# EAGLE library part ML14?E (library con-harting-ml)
HARTING
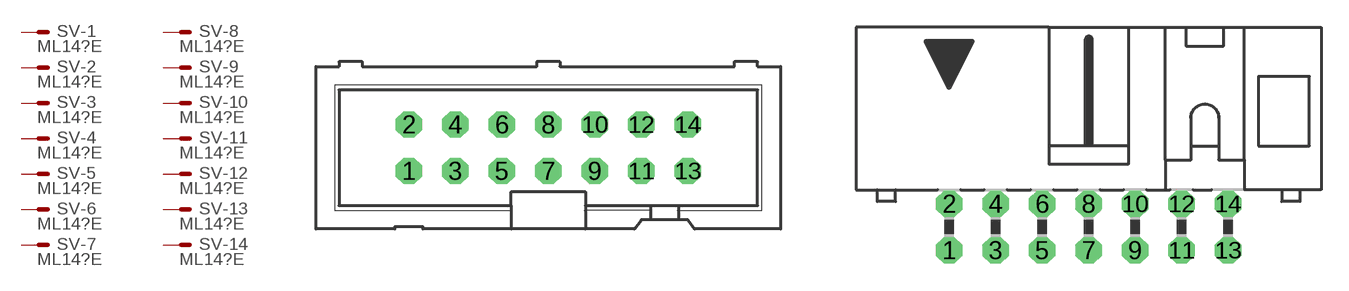
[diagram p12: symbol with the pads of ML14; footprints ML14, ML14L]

Designator prefix SV; gates -1=M -2=M -3=M -4=M -5=M -6=M -7=M -8=M -9=M -10=M -11=M -12=M -13=M -14=M

## ML14E (OC_FARNELL: unknown; OC_NEWARK: unknown)  [ML14]
1  -1:S  pas
2  -2:S  pas
3  -3:S  pas
4  -4:S  pas
5  -5:S  pas
6  -6:S  pas
7  -7:S  pas
8  -8:S  pas
9  -9:S  pas
10  -10:S  pas
11  -11:S  pas
12  -12:S  pas
13  -13:S  pas
14  -14:S  pas

## ML14LE (OC_FARNELL: unknown; OC_NEWARK: unknown)  [ML14L]
Pads as for ML14

## ML143ME (OC_FARNELL: unknown; OC_NEWARK: unknown)  [3M_14]
Pads as for ML14

## ML143MLE (OC_FARNELL: unknown; OC_NEWARK: unknown)  [3M_14L]
Pads as for ML14

## Footprint ML14 (pad centres in mm)
HARTING
drill 0.914 octagon: 1 -7.62,-1.27; 2 -7.62,1.27; 3 -5.08,-1.27; 4 -5.08,1.27; 5 -2.54,-1.27; 6 -2.54,1.27; 7 0,-1.27; 8 0,1.27; 9 2.54,-1.27; 10 2.54,1.27; 11 5.08,-1.27; 12 5.08,1.27; 13 7.62,-1.27; 14 7.62,1.27

## Footprint ML14L (pad centres in mm)
HARTING
drill 0.914 octagon: 1 -7.62,-1.27; 2 -7.62,1.27; 3 -5.08,-1.27; 4 -5.08,1.27; 5 -2.54,-1.27; 6 -2.54,1.27; 7 0,-1.27; 8 0,1.27; 9 2.54,-1.27; 10 2.54,1.27; 11 5.08,-1.27; 12 5.08,1.27; 13 7.62,-1.27; 14 7.62,1.27

## Footprint 3M_14 (pad centres in mm)
3M
drill 0.813 square: 1 -7.62,-1.27; 2 -7.62,1.27; 3 -5.08,-1.27; 4 -5.08,1.27; 5 -2.54,-1.27; 6 -2.54,1.27; 7 0,-1.27; 8 0,1.27; 9 2.54,-1.27; 10 2.54,1.27; 11 5.08,-1.27; 12 5.08,1.27; 13 7.62,-1.27; 14 7.62,1.27

## Footprint 3M_14L (pad centres in mm)
3M
drill 0.813 square: 1 -7.62,-5.08; 2 -7.62,-2.54; 3 -5.08,-5.08; 4 -5.08,-2.54; 5 -2.54,-5.08; 6 -2.54,-2.54; 7 0,-5.08; 8 0,-2.54; 9 2.54,-5.08; 10 2.54,-2.54; 11 5.08,-5.08; 12 5.08,-2.54; 13 7.62,-5.08; 14 7.62,-2.54
hole 2.54 at -13.538,-3.277
hole 2.54 at 13.538,-3.277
